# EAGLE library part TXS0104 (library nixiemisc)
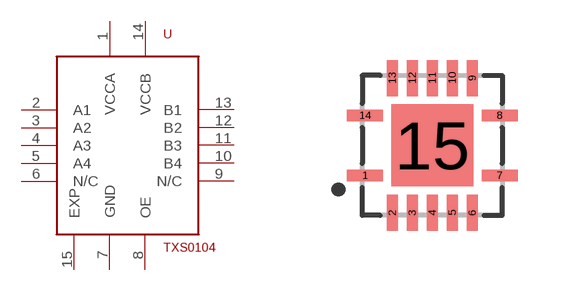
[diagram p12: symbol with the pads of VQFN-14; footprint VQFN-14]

Designator prefix U

## TXS0104  [VQFN-14]
1  VCCA  pwr
2  A1  pas
3  A2  pas
4  A3  pas
5  A4  pas
6  N/C  nc
7  GND  pwr
8  OE  pas
9  N/C  nc
10  B4  pas
11  B3  pas
12  B2  pas
13  B1  pas
14  VCCB  pwr
15  EXP  pwr

## Footprint VQFN-14 (pad centres in mm)
smd 0.9 x 0.28: 1 -1.685,-0.75; 7 1.685,-0.75; 8 1.685,0.75; 14 -1.685,0.75
smd 0.28 x 0.9: 2 -1,-1.685; 3 -0.5,-1.685; 4 0,-1.685; 5 0.5,-1.685; 6 1,-1.685; 9 1,1.685; 10 0.5,1.685; 11 0,1.685; 12 -0.5,1.685; 13 -1,1.685
smd 2.05 x 2.05: 15 0,0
